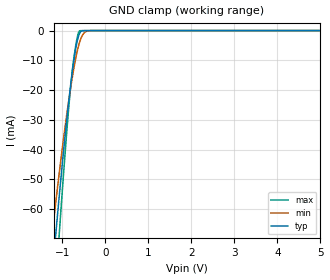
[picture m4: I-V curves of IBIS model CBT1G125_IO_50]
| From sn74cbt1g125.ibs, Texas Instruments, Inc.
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[Model]   CBT1G125_IO_50
Model_type  Terminator
| variable   typ   min   max
C_comp   3.53pF   2.80pF   7.34pF
| C_tri-state   3.53pF   2.80pF   7.34pF
[Temperature Range]   40   100   -40
| Ambient temperature   25   85   -40
[Voltage range]   5   4.5   5.5
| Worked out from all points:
|   GND clamp passes 1 mA (typ) near -0.60 V on its own axis
[GND Clamp]
| CBT1G125_IO_50
|   Voltage   I(typ)   I(min)   I(max)
-5V       -850.7mA   -691.8mA   -1.075A
-1.235V   -82.79mA   -68.78mA   -104.6mA
-1.155V   -69.58mA   -58.6mA    -87.07mA
-1.075V   -56.82mA   -48.79mA   -70.04mA
-1.04V    -51.4mA    -44.64mA   -62.79mA
-895mV    -30.29mA   -28.47mA   -34.45mA
-790mV    -16.86mA   -18.11mA   -17.04mA
-680mV    -5.731mA   -9.023mA   -4.668mA
-595mV    -970.9uA   -3.956mA   -98.27uA
-485mV    -32.41uA   -710.3uA   -822.3nA
-330mV    -247.2nA   -18.46uA   -1.711nA
5V        53.08pA    2.956nA    25.73pA
